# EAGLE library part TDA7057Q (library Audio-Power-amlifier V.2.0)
The TDA7057Q is a stereo output amplifier in a 13 pin power package. The device is designed for battery-fed portable stereo recorders and radios, but also suitable for mains-fed applications.
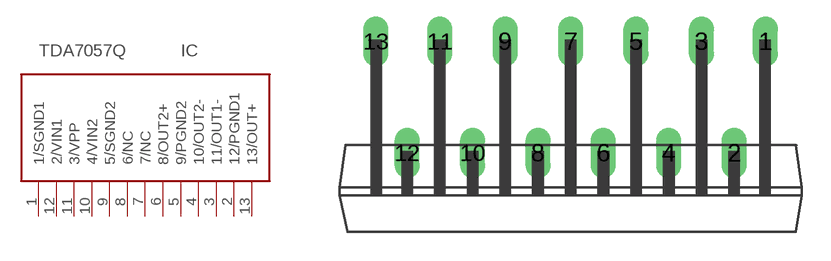
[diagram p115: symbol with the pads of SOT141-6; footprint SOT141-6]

Designator prefix IC

## TDA7057QDBS13P  [SOT141-6]
1  1/SGND1  pwr
2  12/PGND1  pwr
3  11/OUT1-  out
4  10/OUT2-  out
5  9/PGND2  pwr
6  8/OUT2+  out
7  7/NC  nc
8  6/NC  nc
9  5/SGND2  pwr
10  4/VIN2  in
11  3/VPP  pwr
12  2/VIN1  in
13  13/OUT+  out

## Footprint SOT141-6 (pad centres in mm)
drill 0.8 long: 1 10.12,5.8; 2 8.5,0; 3 6.8,5.8; 4 5.1,0; 5 3.4,5.8; 6 1.7,0; 7 0,5.8; 8 -1.7,0; 9 -3.4,5.8; 10 -5.1,0; 11 -6.8,5.8; 12 -8.5,0; 13 -10.12,5.8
